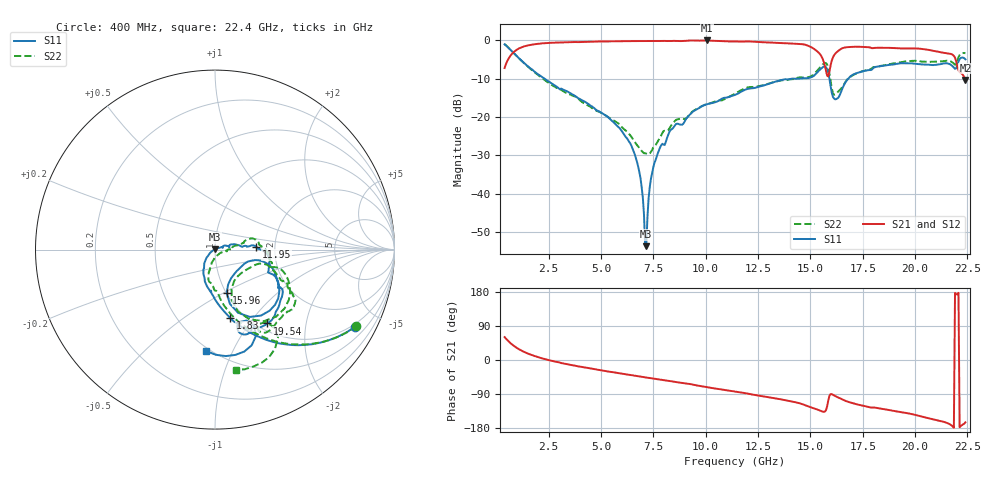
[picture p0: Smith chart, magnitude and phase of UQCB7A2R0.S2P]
!  Part Number  UQCB7A2R0	Mounting Orientation: Vertical
!  Description: RF capacitors
!  Application: Coupling, Bypass, Tuning, DC Block
!  Filters, Matching
# GHZ S DB R 50
! Freq  |S11|  S11 Ph  |S21|  S21 Ph  |S12|  S12 Ph  |S22|  S22 Ph
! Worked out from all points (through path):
!   401 points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, 400 MHz to 22.4 GHz, reference 50 ohm
!   highest |S21| = 0.00 dB at 10.08 GHz (marker M1); lowest = -10.3 dB at 22.4 GHz (marker M2)
!   group delay of S21, straight-line fit = 23.9 ps
!   lowest |S11| = -53.7 dB at 7.165 GHz (marker M3), VSWR 1.00, Z = 50.1 + j0.193 ohm
!   |S11| at or under -10 dB: 2.304 GHz to 14.1 GHz (11.79 GHz wide, 144 % of centre); 14.315 GHz to 14.315 GHz (0 Hz wide, 0 % of centre); 15.91 GHz to 16.8 GHz (895.1 MHz wide, 5.47 % of centre)
!   |S22| runs from -29.7 to -1.0 dB; largest |S21 - S12| = 0.0043
!   S11 on the Smith chart (normalised r, x): 400 MHz: 0.89, -3.68; 1.83 GHz: 0.86, -0.78; 11.95 GHz: 1.60, +0.05; 15.96 GHz: 1.00, -0.52; 19.54 GHz: 1.11, -1.23; 22.4 GHz: 0.48, -0.79
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0.4  -1.01 -28.9  -7.18 60.4  -7.16 60.4  -0.96 -28.5
1.06  -4.51 -58.9  -2.17 29.3  -2.15 29.2  -4.51 -58.0
1.83  -8.15 -77.4  -0.99 10.5  -0.96 10.5  -8.31 -75.1
4.085  -15.59 -110.7  -0.39 -18.3  -0.37 -18.4  -16.03 -103.3
6.395  -26.82 -140.9  -0.18 -39.4  -0.17 -39.6  -24.74 -98.6
6.78  -33.03 -150.1  -0.15 -42.9  -0.15 -43.0  -27.70 -84.4
7.165  -53.72 69.6  -0.15 -46.2  -0.15 -46.4  -29.56 -54.4
7.44  -34.65 27.0  -0.15 -48.6  -0.16 -48.8  -28.62 -26.6
7.77  -28.66 20.8  -0.14 -51.3  -0.15 -51.5  -25.83 -9.6
10.08  -16.64 6.8  0.00 -71.7  -0.02 -71.9  -16.66 11.4
11.4  -14.23 5.7  -0.25 -83.5  -0.25 -83.6  -13.96 17.1
11.95  -12.73 3.8  -0.26 -88.1  -0.26 -88.2  -12.35 11.7
15.085  -9.49 -23.3  -1.89 -126.1  -1.91 -126.1  -9.17 -16.4
15.69  -6.81 -48.2  -6.61 -136.1  -6.62 -136.0  -5.89 -40.1
15.965  -11.96 -75.0  -6.49 -90.0  -6.55 -90.2  -10.60 -71.5
16.185  -15.38 -44.9  -3.46 -95.4  -3.48 -95.3  -14.11 -41.0
16.57  -12.02 -13.8  -1.94 -105.3  -1.95 -105.3  -11.76 -17.6
18.77  -6.37 -43.3  -1.93 -132.2  -1.96 -132.1  -6.19 -29.2
19.54  -5.95 -54.7  -2.08 -139.4  -2.10 -139.3  -5.48 -32.8
21.685  -6.28 -73.4  -3.50 -170.6  -3.50 -170.5  -5.41 -59.8
22.07  -5.48 -64.6  -7.81 177.3  -7.84 177.7  -4.39 -54.4
22.4  -4.93 -95.1  -10.30 -164.4  -10.32 -164.5  -3.34 -80.3
